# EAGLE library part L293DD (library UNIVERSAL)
4X 600mA half bridge driver.
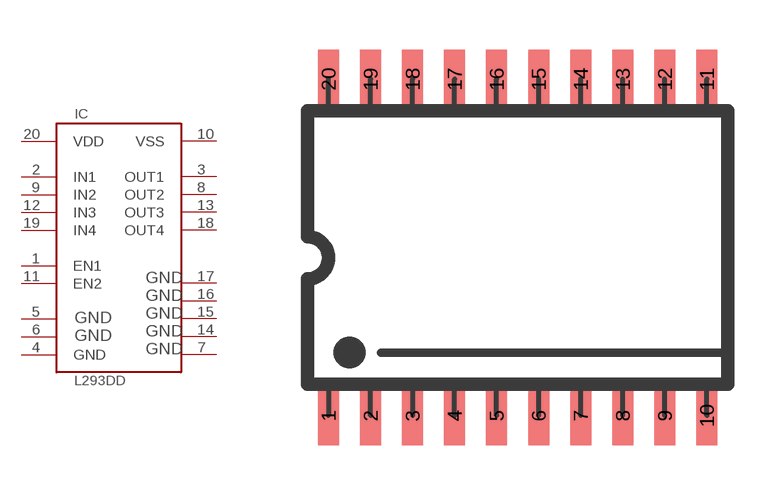
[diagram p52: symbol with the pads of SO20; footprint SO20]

Designator prefix IC

## L293DD  [SO20]
1  EN1  in
2  IN1  in
3  OUT1  out
4  GND  pwr
5  GND1  pwr
6  GND2  pwr
7  GND3  pwr
8  OUT2  out
9  IN2  in
10  VSS  pwr
11  EN2  in
12  IN3  in
13  OUT3  out
14  GND4  pwr
15  GND5  pwr
16  GND6  pwr
17  GND7  pwr
18  OUT4  out
19  IN4  in
20  VDD  pwr

## Footprint SO20 (pad centres in mm)
smd 0.635 x 1.778: 1 0,0; 2 1.27,0; 3 2.54,0; 4 3.81,0; 5 5.08,0; 6 6.35,0; 7 7.62,0; 8 8.89,0; 9 10.16,0; 10 11.43,0; 11 11.43,10.16; 12 10.16,10.16; 13 8.89,10.16; 14 7.62,10.16; 15 6.35,10.16; 16 5.08,10.16; 17 3.81,10.16; 18 2.54,10.16; 19 1.27,10.16; 20 0,10.16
